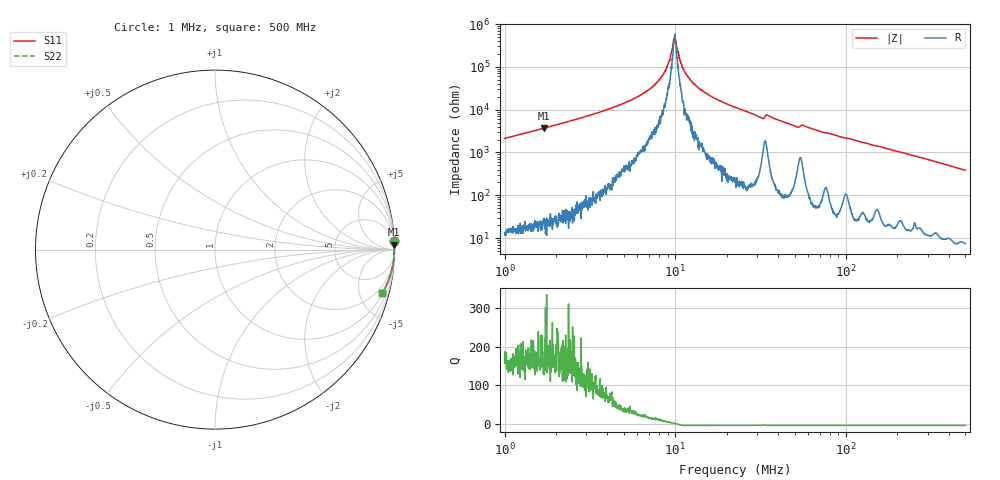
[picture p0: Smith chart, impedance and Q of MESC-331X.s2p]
!s-Parameter Generated by FASTRON Sdn. Bhd.
!FASTRON P/N : MESC-331X
!Keysight Technologies,E4991B,MY54100416,A.01.15
!Date: Fri Mar 27 11:30:20 2026
!Version  : Rev00 Fri Mar 27 11:30:20 2026
!Data & Calibration Information:
!PortZ  Port1:50+j0  Port2:50+j0
!When reading, reference impedance value at option line is always used.
! Remarks : This data is being provided solely for informational purposes.
!Freq	S11	S21	S12	S22
# Hz S dB R 50
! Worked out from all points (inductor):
!   1601 points, 1 MHz to 500 MHz, reference 50 ohm
!   read as one part in series: L = 336 uH near 1.032 MHz
!   highest Q = 201 at 1.709 MHz (marker M1), where L = 346 uH
!   self-resonance near 9.853 MHz
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1000000  -0.01 2.7  -26.58 -86.9  -26.58 -86.9  -0.01 2.7
1709174  -0.00 1.5  -31.40 -88.1  -31.40 -88.1  -0.00 1.5
2820919  -0.00 0.9  -36.24 -88.7  -36.24 -88.7  -0.00 0.9
5480788  -0.00 0.3  -44.38 -88.0  -44.38 -88.0  -0.00 0.3
6812507  -0.00 0.2  -48.78 -86.2  -48.78 -86.2  -0.00 0.2
7957584  -0.00 0.1  -53.51 -83.9  -53.51 -83.9  -0.00 0.1
8906356  -0.00 0.1  -60.06 -78.5  -60.06 -78.5  -0.00 0.1
9331304  -0.00 0.0  -64.05 -71.7  -64.05 -71.7  -0.00 0.0
9700875  -0.00 0.0  -70.06 -46.8  -70.06 -46.8  -0.00 0.0
9968250  -0.00 -0.0  -73.64 11.7  -73.64 11.7  -0.00 -0.0
1.073172e7  -0.00 -0.0  -62.55 74.7  -62.55 74.7  -0.00 -0.0
1.11135e7  -0.00 -0.1  -59.15 80.3  -59.15 80.3  -0.00 -0.1
1.263331e7  -0.00 -0.1  -52.61 85.8  -52.61 85.8  -0.00 -0.1
1.60732e7  -0.00 -0.3  -46.41 87.8  -46.41 87.8  -0.00 -0.3
2.236068e7  -0.00 -0.5  -41.10 88.5  -41.10 88.5  -0.00 -0.5
3.196508e7  -0.01 -0.9  -36.07 83.8  -36.07 83.8  -0.01 -0.9
3.495212e7  -0.01 -0.8  -37.30 83.1  -37.30 83.1  -0.01 -0.8
5.11429e7  -0.02 -1.4  -32.06 84.4  -32.06 84.4  -0.02 -1.4
5.592205e7  -0.02 -1.3  -32.69 83.2  -32.69 83.2  -0.02 -1.3
6.307767e7  -0.01 -1.6  -31.07 87.3  -31.07 87.3  -0.01 -1.6
1.77937e8  -0.04 -4.8  -21.62 84.2  -21.62 84.2  -0.04 -4.8
5e8  -0.33 -14.6  -11.97 74.3  -11.97 74.3  -0.33 -14.6
